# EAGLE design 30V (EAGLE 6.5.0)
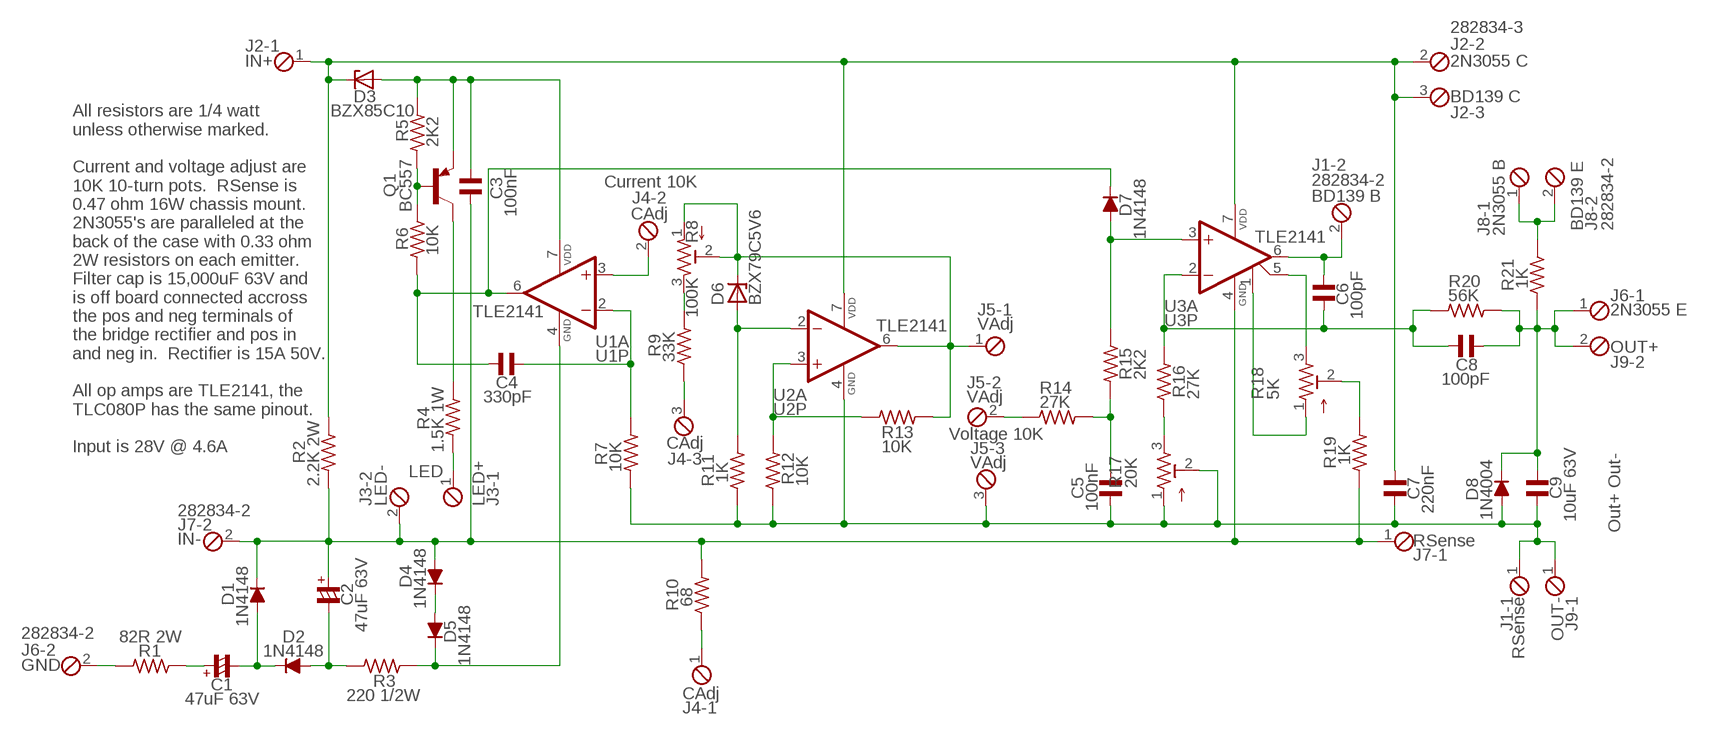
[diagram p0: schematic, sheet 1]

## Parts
C1  47uF 63V  CPOL-USE5-6  [E5-6]
C2  47uF 63V  CPOL-USE5-6  [E5-6]
C3  100nF  C5/2.5  [C5B2.5]
C4  330pF  C-US050-024X044  [C050-024X044]
C5  100nF  C5/2.5  [C5B2.5]
C6  100pF  C-US050-024X044  [C050-024X044]
C7  220nF  C5/3.5  [C5B3.5]
C8  100pF  C-US050-024X044  [C050-024X044]
C9  10uF 63V  C22/8  [C22.5B8]
D1  1N4148  [DO35-10]
D2  1N4148  [DO35-10]
D3  BZX85C10  ZPD  [DO35Z10]
D4  1N4148  [DO35-10]
D5  1N4148  [DO35-10]
D6  BZX79C5V6  ZPD  [DO35Z10]
D7  1N4148  [DO35-10]
D8  1N4004  [DO41-10]
J1  282834-2  [282834-2]
J2  282834-3  [282834-3]
J3  LED  282834-2  [282834-2]
J4  Current 10K  282834-3  [282834-3]
J5  Voltage 10K  282834-3  [282834-3]
J6  282834-2  [282834-2]
J7  282834-2  [282834-2]
J8  282834-2  [282834-2]
J9  Out+ Out-  282834-2  [282834-2]
Q1  BC557  MPSA56-TO92  [TO92-CBE]
R1  82R 2W  R-US_0411/15  [0411/15]
R2  2.2K 2W  R-US_0411/15  [0411/15]
R3  220 1/2W  R-US_0309/12  [0309/12]
R4  1.5K 1W  R-US_0411/15  [0411/15]
R5  2K2  R-US_0207/10  [0207/10]
R6  10K  R-US_0207/10  [0207/10]
R7  10K  R-US_0207/10  [0207/10]
R8  100K  TRIM_US-3296W  [3296W]
R9  33K  R-US_0207/10  [0207/10]
R10  68  R-US_0207/10  [0207/10]
R11  1K  R-US_0207/10  [0207/10]
R12  10K  R-US_0207/10  [0207/10]
R13  10K  R-US_0207/10  [0207/10]
R14  27K  R-US_0207/10  [0207/10]
R15  2K2  R-US_0207/10  [0207/10]
R16  27K  R-US_0207/10  [0207/10]
R17  20K  TRIM_US-3296W  [3296W]
R18  5K  TRIM_US-3296W  [3296W]
R19  1K  R-US_0207/10  [0207/10]
R20  56K  R-US_0207/10  [0207/10]
R21  1K  R-US_0207/10  [0207/10]
U1  TLE2141  TLC080P  [DIL08]
U2  TLE2141  TLC080P  [DIL08]
U3  TLE2141  TLC080P  [DIL08]

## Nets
N$1: J6.2 R1.2
N$2: C6.2 C8.2 R16.2 R20.1 U3.2(-IN)
N$3: C7.1 D3.C J2.1 J2.2 J2.3 R2.2 U2.7(VDD) U3.7(VDD)
N$4: C2.+ C3.2 D1.C D4.A J3.2 J7.1 J7.2 R2.1 R10.1 R19.1 U3.4(GND)
N$5: J3.1 R4.1
N$6: R8.3 R9.2
N$7: D4.C D5.A
N$8: D5.C R3.2 U1.4(GND)
N$9: C2.- D2.A R3.1
N$10: C1.+ R1.1
N$11: C1.- D1.A D2.C
N$12: R18.1 U3.1(NULL1)
N$13: R16.1 R17.3
N$14: Q1.C R4.2
N$15: C3.1 D3.A Q1.E R5.2 U1.7(VDD)
N$16: Q1.B R5.1 R6.2
N$17: C4.2 D7.C R6.1 U1.6(OUT)
N$18: R18.3 U3.5(NULL2)
N$19: C4.1 R7.2 U1.2(-IN)
N$20: J4.2 U1.3(+IN)
N$21: D6.A R11.2 U2.2(-IN)
N$22: C6.1 J1.2 U3.6(OUT)
N$23: J4.1 R10.2
N$24: R12.2 R13.1 U2.3(+IN)
N$25: R18.2 R19.2
N$26: C8.1 C9.2 D8.C J6.1 J9.2 R20.2 R21.2
N$27: J4.3 R9.1
N$28: D6.C J5.1 R8.1 R8.2 R13.2 U2.6(OUT)
N$31: J8.1 J8.2 R21.1
N$32: J5.2 R14.1
N$33: C5.1 R14.2 R15.1
N$34: D7.A R15.2 U3.3(+IN)
N$36: C5.2 C7.2 C9.1 D8.A J1.1 J5.3 J9.1 R7.1 R11.1 R12.1 R17.1 R17.2 U2.4(GND)
Unconnected: U1.1(NULL1) U1.5(NULL2) U1.8(SHDN) U2.1(NULL1) U2.5(NULL2) U2.8(SHDN) U3.8(SHDN)

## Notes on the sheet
- IN+ | 2N3055 C
- BD139 C
- BD139 B
- CAdj
- BD139 E
- 2N3055 B
- 2N3055 E
- VAdj
- OUT+
- VAdj
- CAdj
- All resistors are 1/4 watt
  unless otherwise marked.
  
  Current and voltage adjust are
  10K 10-turn pots.  RSense is
  0.47 ohm 16W chassis mount.
  2N3055's are paralleled at the
  back of the case with 0.33 ohm
  2W resistors on each emitter.
  Filter cap is 15,000uF 63V and
  is off board connected accross
  the pos and neg terminals of
  the bridge rectifier and pos in
  and neg in.  Rectifier is 15A 50V.
  
  All op amps are TLE2141, the
  TLC080P has the same pinout.
  
  Input is 28V @ 4.6A
- VAdj
- LED- | LED+
- IN- | RSense
- RSense | OUT-
- GND
- CAdj

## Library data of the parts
C1 C2 = rcl:CPOL-US: POLARIZED CAPACITOR, American symbol
C3 C5 C7 C9 = capacitor-wima:C: CAPACITOR
C4 C6 C8 = rcl:C-US: CAPACITOR, American symbol
D1 D2 D4 D5 D7 = diode:1N4148: DIODE
D3 D6 = diode:ZPD: Z DIODE
D8 = diode:1N4004: DIODE
J1 J3 J6-J9 = con-tyco:282834-2: TERMINAL BLOCK
J2 J4 J5 = con-tyco:282834-3: TERMINAL BLOCK
Q1 = transistor-pnp:*-?: PNP Transistor
R1-R7 R9-R16 R19-R21 = rcl:R-US_: RESISTOR, American symbol
R8 R17 R18 = pot:TRIM_US-: POTENTIOMETER
U1-U3 = op-amp:TLC080: BiMOS OP-AMP Single Supply, External Shutdown

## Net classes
0 default: clearance 0.205 mm

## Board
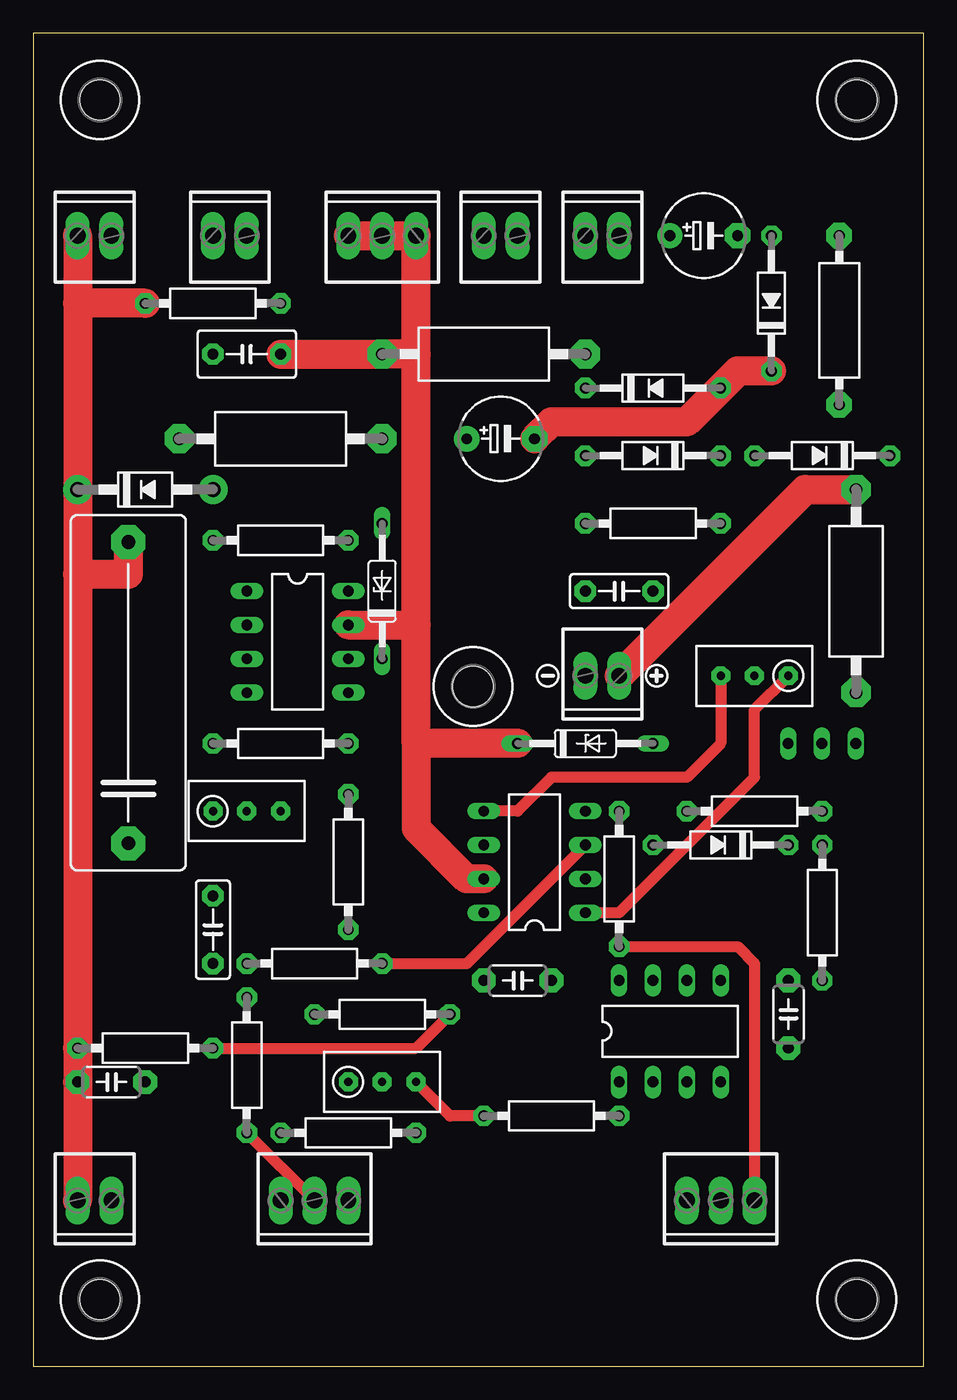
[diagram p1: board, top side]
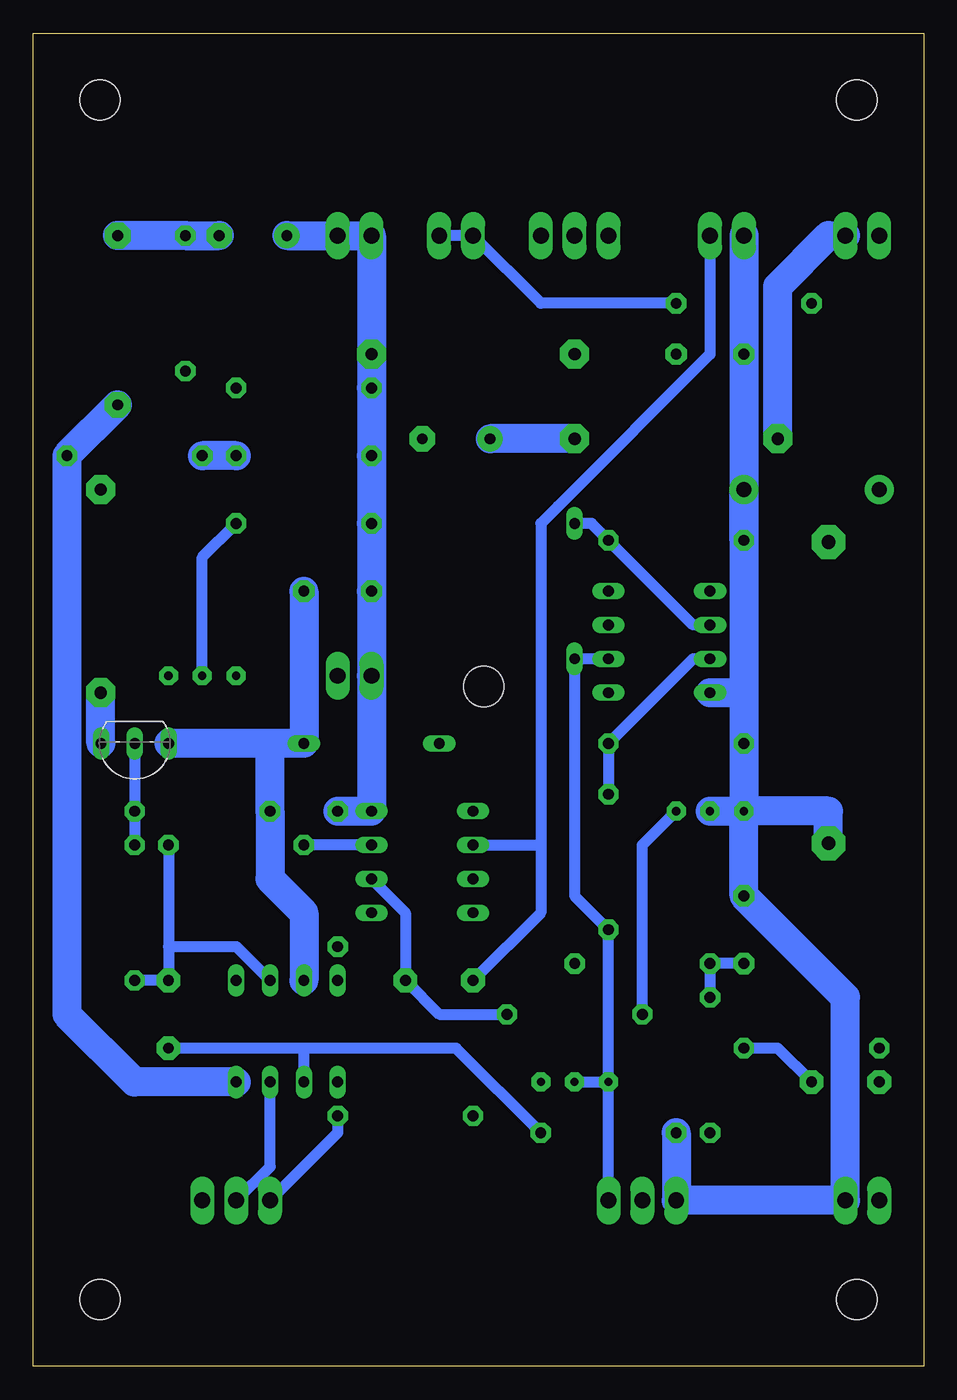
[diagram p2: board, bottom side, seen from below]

Size 66.8 x 100 mm. Coordinates in mm from the lower left corner, seen from the top.
Outline: 0,0 66.8,0 66.8,100 0,100 0,0
Copper layers (1*2*15*16): Top 0.035mm / dielectric 0.2mm / Route2 0.0175mm / dielectric 1.1mm / Route15 0.0175mm / dielectric 0.2mm / Bottom 0.035mm
Design rules "SeeedStudio_DRU_no_angle_20130527 *": minimum track width 6mil, minimum drill 12mil, track to track 6mil, track to pad 6mil, pad to pad 6mil, via to via 6mil, smd to smd 0mil, copper to edge 10mil, drill to drill 10mil, minimum pad ring 6mil, minimum via ring 6mil, stop-mask expansion 2mil, vias tented up to drill 25mil, thermal gap 10mil

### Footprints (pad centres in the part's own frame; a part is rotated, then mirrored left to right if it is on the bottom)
E5-6 = drill 0.813 pad 1.905: + -2.54,0 | drill 0.813 pad 1.905 octagon: - 2.54,0
C5B2.5 = drill 0.813 pad 1.6 octagon: 1 -2.54,0; 2 2.54,0
C050-024X044 = drill 0.813 pad 1.778 octagon: 1 -2.54,0; 2 2.54,0
C5B3.5 = drill 0.813 pad 1.6 octagon: 1 -2.54,0; 2 2.54,0
C22.5B8 = drill 1.016 pad 2.54 octagon: 1 -11.303,0; 2 11.303,0
DO35-10 = drill 0.813 pad 1.524 octagon: A 5.08,0; C -5.08,0
DO35Z10 = drill 0.813 long: A 5.08,0; C -5.08,0
DO41-10 = drill 1.118 pad 2.184: A 5.08,0; C -5.08,0
282834-2 = drill 1.194 long: 1 -1.27,0; 2 1.27,0
282834-3 = drill 1.194 long: 1 -2.54,0; 2 0,0; 3 2.54,0
TO92-CBE = drill 0.813 long: B 0,0; C 2.54,0; E -2.54,0
0411/15 = drill 0.914 pad 2.184 octagon: 1 -7.62,0; 2 7.62,0
0309/12 = drill 0.813 pad 1.93 octagon: 1 -6.35,0; 2 6.35,0
0207/10 = drill 0.813 pad 1.524 octagon: 1 -5.08,0; 2 5.08,0
3296W = drill 0.61 pad 1.422 octagon: 1 0,-2.54; 2 0,0; 3 0,2.54
DIL08 = drill 0.813 long: 1 -3.81,-3.81; 2 -1.27,-3.81; 3 1.27,-3.81; 4 3.81,-3.81; 5 3.81,3.81; 6 1.27,3.81; 7 -1.27,3.81; 8 -3.81,3.81
120 = hole 3.048: 0,0

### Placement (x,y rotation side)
C1  35.07,69.58 0 top
C2  50.31,84.82 0 top
C3  43.96,58.15 180 top
C4  56.66,26.4 90 top
C5  13.48,32.75 90 top
C6  36.34,28.94 0 top
C7  16.02,75.93 180 top
C8  5.86,21.32 0 top
C9  7.13,50.53 90 top
D1  46.5,73.39 0 top
D2  55.39,79.74 90 top
D3  41.42,46.72 0 top
D4  46.5,68.31 180 top
D5  59.2,68.31 180 top
D6  26.18,58.15 90 top
D7  51.58,39.1 180 top
D8  8.4,65.77 0 top
J1  14.75,84.82 0 top
J2  26.18,84.82 0 top
J3  42.69,51.8 180 top
J4  51.58,12.43 180 top
J5  21.1,12.43 180 top
J6  4.59,84.82 0 top
J7  42.69,84.82 0 top
J8  35.07,84.82 0 top
J9  4.59,12.43 180 top
Q1  59.18,46.72 180 bottom
R1  18.56,69.58 180 top
R2  33.8,75.93 180 top
R3  60.47,78.47 270 top
R4  61.74,58.15 270 top
R5  54.12,41.64 180 top
R6  59.2,34.02 90 top
R7  23.64,17.51 0 top
R8  26.18,21.32 270 top
R9  38.88,18.78 180 top
R10  43.96,36.56 270 top
R11  18.56,61.96 0 top
R12  18.56,46.72 0 top
R13  23.64,37.83 270 top
R14  16.02,22.59 90 top
R15  21.1,30.21 0 top
R16  26.18,26.4 0 top
R17  16.02,41.64 270 top
R18  54.12,51.8 90 top
R19  46.5,63.23 0 top
R20  8.4,23.86 180 top
R21  13.48,79.74 180 top
U1  47.77,25.13 0 top
U2  19.83,54.34 270 top
U3  37.61,37.83 90 top
U$1  [120]  5,95 0 top
U$2  [120]  61.8,95 0 top
U$3  [ICON_MINUS]  38.61,51.8 0 top
U$4  [120]  5,5 0 top
U$5  [120]  61.8,5 0 top
U$6  [ICON_PLUS]  46.77,51.8 0 top
U$7  [120]  33,51 0 top

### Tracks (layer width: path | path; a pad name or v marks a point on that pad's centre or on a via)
N$1
  Bottom 2.184: R1.2 10.94,81.01 7.13,84.82 J6.2
N$2
  Top 0.813: R20.1 28.72,23.86 R16.2
  Bottom 0.813: U3.2 38.88,34.02 C6.2 36.34,26.4 R16.2 | C8.2 10.94,23.86 R20.1
N$3
  Top 2.184: 28.72,46.72 28.72,40.37 32.52,36.56 U3.7 | D3.C 28.72,46.72 | C7.1 R2.2 28.72,75.93 | J2.1 J2.2 J2.3 28.72,75.93 | 28.72,46.72 28.72,55.61 | 28.72,55.61 28.72,75.93 | U2.7 28.72,55.61
N$4
  Bottom 2.184: C2.+ J7.2 J7.1 R2.1 D1.C D4.A R19.1 C3.2 J3.2 U3.4 R10.1
N$5
  Top 2.184: J3.1 57.93,65.77 R4.1
N$6
  Top 0.813: R9.2 31.26,18.78 R8.3
N$7
  Bottom 2.184: D4.C D5.A
N$8
  Bottom 2.184: R3.2 D5.C 64.28,26.4 59.2,21.32 U1.4
N$9
  Bottom 2.184: C2.- D2.A R3.1
N$10
  Bottom 2.184: R1.1 C1.+
N$11
  Top 2.184: D2.C 52.85,74.66 D1.A 49.04,70.85 38.87,70.85 C1.-
N$12
  Top 0.813: U3.1 43.96,34.02 54.12,44.18 54.12,49.26 R18.1
N$13
  Bottom 0.813: R16.1 21.1,39.1 R17.3
N$14
  Bottom 2.184: Q1.C 61.74,46.72 R4.2
N$15
  Bottom 2.184: U1.7 46.5,34.02 49.04,36.56 R5.2 49.04,46.72 | 49.04,46.72 D3.A C3.1 | 49.04,46.72 Q1.E
N$16
  Bottom 0.813: Q1.B R5.1 R6.2
N$17
  Bottom 0.813: D7.C 56.66,31.48 | 56.66,31.48 C4.2 R6.1 | 56.66,31.48 51.58,31.48 U1.6
N$18
  Top 0.813: R18.3 51.58,46.72 49.04,44.18 38.88,44.18 36.34,41.64 U3.5
N$19
  Bottom 0.813: 46.5,23.86 C4.1 | U1.2 46.5,23.86 | R7.2 35.07,23.86 46.5,23.86
N$20
  Bottom 0.813: J4.2 49.03,14.97 U1.3
N$21
  Bottom 0.813: U2.2 17.29,55.61 R11.2 24.91,63.23 D6.A
N$22
  Bottom 0.813: 28.72,39.1 28.72,34.02 C6.1 | U3.6 28.72,39.1 | J1.2 16.02,75.93 27.44,64.51 28.71,63.23 28.71,39.1 28.72,39.1
N$23
  Top 0.813: R10.2 52.85,31.48 54.12,30.21 J4.1
N$24
  Bottom 0.813: U2.3 17.29,53.07 R12.2 R13.1
N$25
  Bottom 0.813: R18.2 54.12,60.69 R19.2
N$26
  Top 2.184: 3.32,59.42 D8.C 3.32,79.74 | C9.2 7.13,59.42 3.32,59.42 | 3.32,59.42 R20.2 C8.1 J9.2 | J6.1 3.32,79.74 | R21.2 3.32,79.74
N$27
  Bottom 0.813: R9.1 43.95,17.51 J4.3
N$28
  Bottom 0.813: R8.2 R8.1 | J5.1 R8.1 | R8.1 R13.2 26.18,35.29 D6.C U2.6
N$31
  Bottom 0.813: J8.2 J8.1 28.72,79.74 R21.1
N$32
  Top 0.813: R14.1 J5.2
N$33
  Bottom 0.813: R14.2 R15.1 C5.1
N$34
  Top 0.813: R15.2 32.53,30.21 U3.3
  Bottom 0.813: U3.3 D7.A
N$36
  Bottom 2.184: R7.1 J5.3 J9.1 5.86,27.67 C5.2 R17.1 | R17.2 R17.1 | J1.1 C7.2 R11.1 D8.A 13.48,50.53 | 13.48,50.53 R12.1 R17.1 | U2.4 13.48,50.53 | C9.1 7.13,41.64 R17.1

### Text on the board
tValues: 2N3055 / Emitter | GND | RSense / 0.47 16W | BD139 / Base | 2N3055 / Collector | BD139 / Collector | In+ | 2N3055 / Base | BD139 / Emitter | In- | RSense / 0.47 16W | V Zero | V Cal | C Cal | Out+ | Out- | Voltage 10K | Current 10K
